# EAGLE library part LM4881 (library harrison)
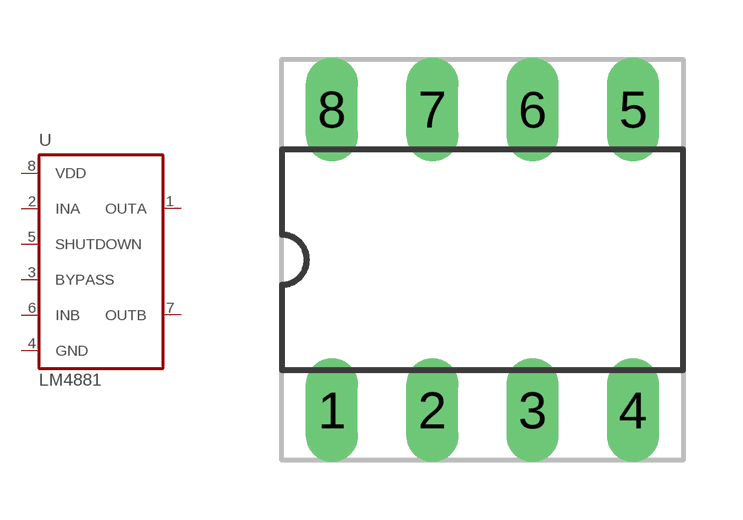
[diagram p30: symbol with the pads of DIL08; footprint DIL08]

Designator prefix U

## LM4881  [DIL08]
1  OUTA  out
2  INA  in
3  BYPASS  pas
4  GND  pwr
5  SHUTDOWN  in
6  INB  in
7  OUTB  out
8  VDD  pwr

## Footprint DIL08 (pad centres in mm)
drill 0.813 long: 1 -3.81,-3.81; 2 -1.27,-3.81; 3 1.27,-3.81; 4 3.81,-3.81; 5 3.81,3.81; 6 1.27,3.81; 7 -1.27,3.81; 8 -3.81,3.81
